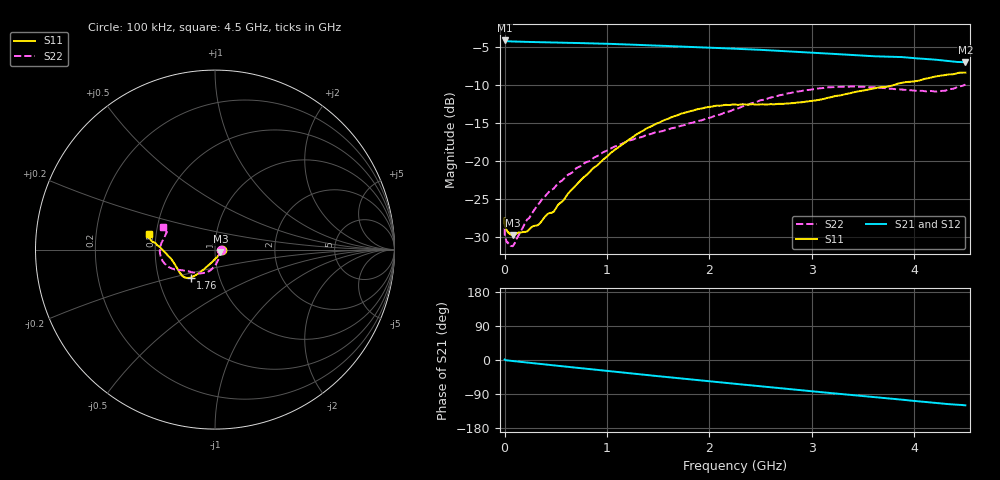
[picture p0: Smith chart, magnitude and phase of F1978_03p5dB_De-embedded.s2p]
! Integrated Device Technology
! Corporate Headquarters
! 6024 Silver Creek Valley Road
! San Jose, CA 95138  USA
! Phone:  1-408-284-8200
! Toll Free:  1-800-223-1366
! Webpage:  http://www.idt.com/
! Timing and RF Division
! 515 Groton Road, Suite 102
! Westford, MA 01886-6024
! Device:  F1978
! Description: 6-bit, 75 ohm, 0.5 dB Digital Step Attenuator
! Frequency:  5.0 MHz -  3.00 GHz
! Package:  4x4 mm QFN Plastic Package: 20 pin
! Ports:  2 RF, 11 DC
!  Pin  1  = D5 (16 dB)
!  Pin  2  = RF1  =  Port 1
!  Pin  3  = Serial Data In (DATA)
!  Pin  4  = Serial Clock (CLK)
!  Pin  5  = Serial Latch Enable (LE)
!  Pin  6  = VDD
!  Pin  7  = NC
!  Pin  8  = NC
!  Pin  9  = NC
!  Pin 10  = GND
!  Pin 11  = GND
!  Pin 12  = NC
!  Pin 13  = VMODE
!  Pin 14  = RF2  =  Port 2
!  Pin 15  = D4 (8 dB)
!  Pin 16  = D3 (4 dB)
!  Pin 17  = D2 (2 dB)
!  Pin 18  = NC
!  Pin 19  = D1 (1 dB)
!  Pin 20  = D0 (0.5 dB)
! State:  7
! Atten State:  3.5 dB
! Voltage:  +3.30 Volts
! Current:  0.565 mA
! Data:  The device was measured on a F1975 evaluation board which has
!  individual transmission lines to the RF pins.  Data was collected
!  using a calibrated network analyzer.  The evaluation board was
!  de-embedded using Automatic Fixture Removal (AFR).
!  The reference plane is the edge of the package pin.
! Misc:
!  Action Tracker AT0416
! Date Measured:  2018-02-08
! Date:  2018-03-26  MJV
! Note:
!  Integrated Device Technology supplies this data as a sample of measured
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# GHz S dB R 75
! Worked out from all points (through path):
!   291 points, 100 kHz to 4.5 GHz, reference 75 ohm
!   highest |S21| = -4.17 dB at 100 kHz (marker M1); lowest = -7.0 dB at 4.5 GHz (marker M2)
!   group delay of S21, straight-line fit = 74.9 ps
!   lowest |S11| = -29.8 dB at 80 MHz (marker M3), VSWR 1.07, Z = 79.6 - j1.89 ohm
!   |S11| at or under -10 dB: start of sweep to 3.812 GHz
!   |S22| runs from -31.3 to -10.0 dB; largest |S21 - S12| = 0.00024
!   S11 on the Smith chart (normalised r, x): 100 kHz: 1.09, +0.00; 1.76 GHz: 0.73, -0.24; 4.5 GHz: 0.45, +0.09
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0.0001  -27.63 0.5  -4.17 1.2  -4.17 1.2  -28.92 0.8
0.001  -28.24 -1.6  -4.20 1.0  -4.20 1.0  -29.61 -1.8
0.003  -28.53 -2.3  -4.22 0.7  -4.22 0.7  -29.92 -2.2
0.017  -29.06 -6.8  -4.26 -0.8  -4.26 -0.8  -30.60 -9.6
0.08  -29.79 -21.5  -4.30 -2.7  -4.30 -2.7  -31.26 -29.4
0.22  -29.33 -45.6  -4.36 -6.8  -4.36 -6.7  -27.76 -56.5
0.36  -28.01 -67.9  -4.40 -10.7  -4.40 -10.7  -25.20 -69.6
0.42  -27.03 -74.3  -4.42 -12.5  -4.42 -12.5  -24.31 -73.5
0.48  -26.71 -82.0  -4.44 -14.1  -4.44 -14.1  -23.67 -77.3
0.76  -22.35 -105.5  -4.52 -22.0  -4.52 -22.1  -20.54 -91.7
1.08  -18.52 -118.0  -4.64 -31.1  -4.64 -31.1  -18.12 -104.8
1.3  -16.44 -123.2  -4.75 -37.3  -4.75 -37.3  -16.98 -113.3
1.52  -14.92 -127.2  -4.86 -43.2  -4.86 -43.2  -16.17 -121.8
1.76  -13.68 -131.1  -4.99 -49.7  -4.99 -49.7  -15.30 -131.6
2.06  -12.77 -137.3  -5.15 -57.7  -5.15 -57.7  -14.04 -142.7
2.26  -12.62 -142.5  -5.26 -63.0  -5.25 -63.0  -13.18 -148.2
2.68  -12.51 -156.3  -5.53 -74.2  -5.53 -74.2  -11.41 -157.6
3.02  -12.11 -167.5  -5.79 -83.1  -5.79 -83.1  -10.58 -166.6
3.4  -11.02 -177.2  -6.09 -92.6  -6.09 -92.6  -10.23 -178.4
3.76  -10.19 176.9  -6.31 -101.3  -6.31 -101.3  -10.52 171.6
4.22  -8.88 171.8  -6.72 -113.6  -6.71 -113.6  -10.89 160.3
4.5  -8.41 167.0  -7.03 -119.6  -7.03 -119.6  -9.98 156.3
